FUNCTION_BLOCK FB 1
TITLE =
//Erste_Schritte_AWL
AUTHOR : Siemens
FAMILY : GetStart
NAME : ENGINE
VERSION : 1.0


VAR_INPUT
  Switch_On : BOOL ;	//Motor einschalten
  Switch_Off : BOOL ;	//Motor ausschalten
  Failure : BOOL ;	//Motorstörung, führt zum Ausschalten
  Actual_Speed : INT ;	//tatsächliche Motordrehzahl
END_VAR
VAR_OUTPUT
  Engine_On : BOOL ;	//Motor wird eingeschaltet
  Preset_Speed_Reached : BOOL ;	//Solldrehzahl erreicht
END_VAR
VAR
  Preset_Speed : INT  := 1500;	//geforderte Motordrehzahl
END_VAR
BEGIN
NETWORK
TITLE =Motor einschalten, Negation von Signalen
//Zum Einschalten des Motors werden die Operationen S (Setzen) und R (Rücksetzen)
//verwendet und so ein speicherndes Verhalten erreicht.
//
//Der Motor wird eingeschaltet, wenn die Variable #Switch_On eingeschaltet ist
//(Signalzustand "1" führt) und die Variable "Automatikbetrieb" ausgeschaltet ist
//(Signalzustand "0" führt). Die Abfrage auf Signalzustand "0" wird durch ein
//nachgestelltes "N" also "UN" dargestellt.
//
//Der Motor wird wieder ausgeschaltet, wenn die Variable #Switch_Off einge-
//schaltet ist oder die Variable #Failure Signalzustand "0" führt. #Failure
//ist ein "nullaktives" Signal, das im Normalfall "1" führt (wenn keine Störung
//ansteht) und im Störfall "0" führt. Auch hier erreichen wir die gewünschte
//Funktionalität, wenn wir das Signal #Failure mit "ON" auf Signalzustand "0"
//abfragen.
//
//Hinweis: "Bausteinlokale" Variablen werden mit #name dargestellt; sie sind nur
//im Baustein "gültig". Globale Variablen "name" stehen in Anführungszeichen; sie
//sind im gesamten Programm "gültig".
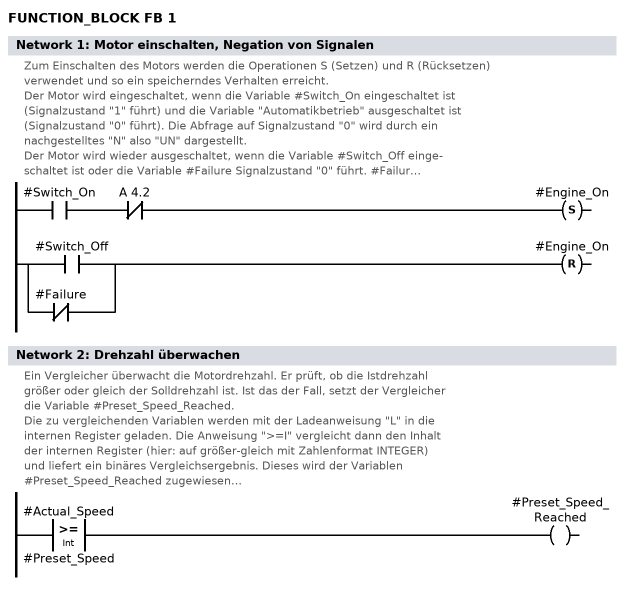
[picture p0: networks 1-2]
      U     #Switch_On;
      UN    A      4.2;
      S     #Engine_On;
      O     #Switch_Off;
      ON    #Failure;
      R     #Engine_On;
NETWORK
TITLE =Drehzahl überwachen
//Ein Vergleicher überwacht die Motordrehzahl. Er prüft, ob die Istdrehzahl
//größer oder gleich der Solldrehzahl ist. Ist das der Fall, setzt der Vergleicher
//die Variable #Preset_Speed_Reached.
//
//Die zu vergleichenden Variablen werden mit der Ladeanweisung "L" in die
//internen Register geladen. Die Anweisung ">=I" vergleicht dann den Inhalt
//der internen Register (hier: auf größer-gleich mit Zahlenformat INTEGER)
//und liefert ein binäres Vergleichsergebnis. Dieses wird der Variablen
//#Preset_Speed_Reached zugewiesen.
//
//Die Motor-Istdrehzahl ist ein Eingangs-Bausteinparameter (Deklaration "in"),
//da sie motorspezifisch ist. Auch die Solldrehzahl ist motorspezifisch; da sie
//jedoch ein fester Wert ist, kann sie statisch in den Motordaten gespeichert
//werden (Deklaration "stat"). Man spricht hier von "statischen Lokalvariablen".
      L     #Actual_Speed;
      L     #Preset_Speed;
      >=I   ;
      =     #Preset_Speed_Reached;
END_FUNCTION_BLOCK

